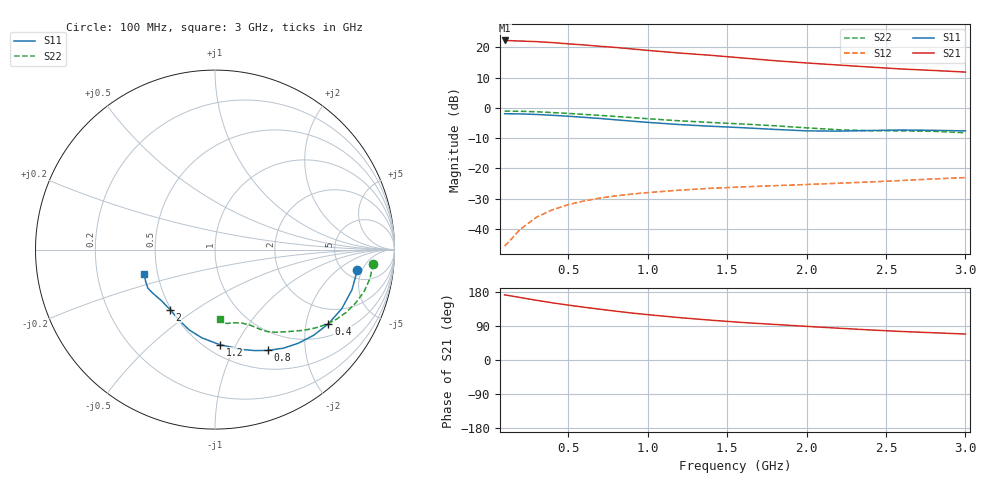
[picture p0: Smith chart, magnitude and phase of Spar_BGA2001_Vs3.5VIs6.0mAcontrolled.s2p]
! Filename: 3_56G1.001
! Title: BGA2001 X0297-20 HFE=80
! Bias: Vce=3.5V; Ic=6.0mA controlled / noise data included
! Company: NXP Semiconductors NL
! User: Quality&Reliability T&D
! Measure time: 23 Oct 1998 / 08:34:12
#  MHz  S  MA  R 50
! Freq  S11  S21  S12  S22  :
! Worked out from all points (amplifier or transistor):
!   20 points, 100 MHz to 3 GHz, reference 50 ohm
!   highest |S21| = 22.3 dB at 100 MHz (marker M1)
!   |S21| within 3 dB of that: start of sweep to 942.5 MHz
!   unconditionally stable (mu >= 1): 1.917 GHz to end of sweep
!   at 400 MHz: K = 0.29, MSG = 27.6 dB, |S12| = -33.7 dB
!   at 1.2 GHz: K = 0.64, MSG = 22.7 dB, |S12| = -27.2 dB
!   at 3 GHz: K = 1.25, MAG = 14.4 dB, |S12| = -23.0 dB
!   lowest NFmin = 1.36 dB at 1.8 GHz
!   S11 on the Smith chart (normalised r, x): 100 MHz: 6.41, -4.08; 400 MHz: 1.40, -2.69; 800 MHz: 0.74, -1.39; 1.2 GHz: 0.59, -0.86; 2 GHz: 0.49, -0.40; 3 GHz: 0.42, -0.14
100  0.8011 -8.2  12.99 171.9  0.005201 68.5  0.8838 -5.1
200  0.7953 -16.4  12.7 164.8  0.009944 77.1  0.8789 -10.3
300  0.7792 -25.0  12.43 157.6  0.01561 76.5  0.8628 -15.8
400  0.755 -33.2  11.99 151.0  0.02071 73.0  0.8377 -20.9
500  0.7282 -40.9  11.43 144.9  0.02519 69.3  0.8106 -25.5
600  0.6982 -48.4  10.95 139.2  0.02902 66.0  0.7813 -29.7
700  0.6684 -55.3  10.41 134.0  0.0324 63.3  0.7518 -33.3
800  0.6351 -62.1  9.95 128.8  0.03523 60.8  0.7216 -36.7
900  0.6049 -68.5  9.416 124.0  0.03768 58.9  0.6919 -39.8
1000  0.5763 -74.8  8.91 119.7  0.03991 57.3  0.6632 -42.8
1200  0.5305 -87.1  8.055 111.8  0.04371 55.0  0.612 -48.3
1400  0.4974 -98.4  7.377 105.0  0.047 53.6  0.5738 -53.4
1600  0.4701 -107.8  6.665 98.9  0.04955 53.3  0.5413 -57.5
1800  0.4412 -116.9  6.017 93.8  0.05191 54.2  0.5068 -60.8
2000  0.4176 -126.9  5.524 88.8  0.0543 54.4  0.4678 -64.6
2200  0.4127 -137.1  5.105 83.9  0.05694 54.5  0.4353 -70.0
2400  0.4231 -144.9  4.724 79.3  0.05979 55.2  0.4193 -76.2
2600  0.4312 -150.0  4.385 75.2  0.06323 57.0  0.4173 -80.8
2800  0.426 -154.8  4.15 71.9  0.06707 57.6  0.4101 -83.5
3000  0.4175 -160.8  3.904 68.5  0.07066 58.4  0.3888 -86.2
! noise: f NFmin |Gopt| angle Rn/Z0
900  1.38  0.29  19.5  0.29
1000  1.46  0.27  19  0.27
1800  1.363  0.264  71.28  0.255
2000  1.41  0.23  70.92  0.226
2200  1.524  0.192  80.92  0.218
2400  1.603  0.187  102.8  0.204
